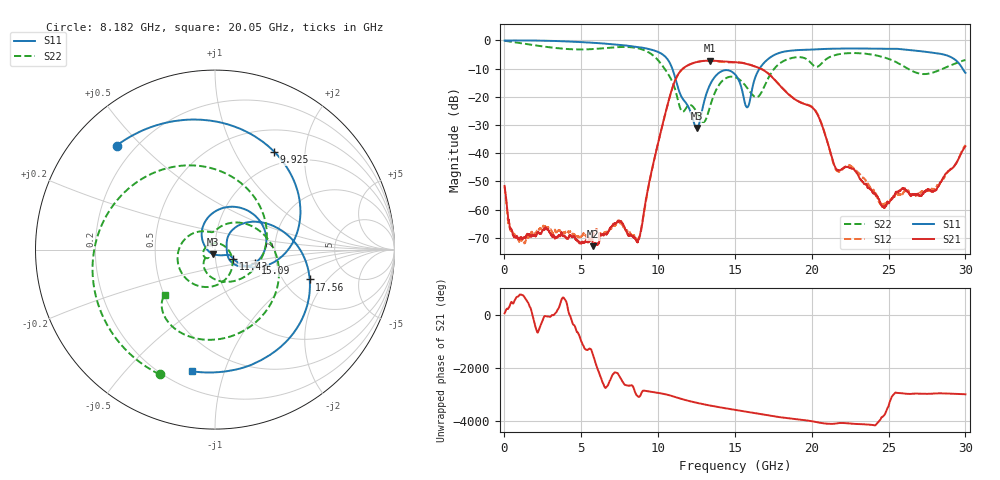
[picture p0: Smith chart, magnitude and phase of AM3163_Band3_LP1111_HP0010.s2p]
!Agilent Technologies,E8364B,MY43040894,A.07.50.67
!Agilent E8364B: A.07.50.67
!Date: Thursday, August 20, 2020 12:15:40
!Correction: S11(Full 2 Port(1,2))
!S21(Full 2 Port(1,2))
!S12(Full 2 Port(1,2))
!S22(Full 2 Port(1,2))
!S2P File: Measurements: S11, S21, S12, S22:
# Hz S  dB  R 50
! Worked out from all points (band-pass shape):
!   3201 points, 10 MHz to 30 GHz, reference 50 ohm
!   highest |S21| = -7.16 dB at 13.38 GHz (marker M1); lowest = -72.9 dB at 5.736 GHz (marker M2)
!   |S21| within 3 dB of the highest: 11.58 GHz to 16.73 GHz (5.157 GHz wide, 36.4 % of centre)
!   lowest |S11| = -31.0 dB at 12.51 GHz (marker M3), VSWR 1.06, Z = 49 - j2.59 ohm
!   |S11| at or under -10 dB: 10.93 GHz to 16.6 GHz (5.674 GHz wide, 41.2 % of centre); 29.81 GHz to end of sweep
!   |S22| runs from -29.0 to -0.1 dB; largest |S21 - S12| = 0.013
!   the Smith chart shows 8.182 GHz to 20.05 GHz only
!   S11 on the Smith chart (normalised r, x): 8.182 GHz: 0.13, +0.42; 9.925 GHz: 0.80, +1.46; 11.43 GHz: 1.22, -0.12; 15.09 GHz: 1.55, -0.25; 17.56 GHz: 2.77, -1.33; 20.05 GHz: 0.30, -0.79
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1e7  -0.04 -2.0  -51.59 49.8  -51.81 -130.8  -0.11 -5.1
1.247088e9  -0.01 -34.1  -70.12 -17.3  -71.29 79.5  -1.12 -82.7
2.652869e9  -0.11 -72.4  -66.44 -54.0  -65.84 103.9  -2.23 -163.0
5.014581e9  -0.60 -135.1  -71.80 53.8  -69.18 113.4  -3.20 71.9
5.736216e9  -0.82 -154.4  -72.94 -31.8  -68.90 -144.7  -3.06 32.0
8.182275e9  -1.96 133.4  -68.85 -162.7  -68.22 59.0  -2.38 -113.9
8.800819e9  -2.41 111.0  -69.56 150.4  -69.26 153.6  -2.91 -157.2
9.925444e9  -3.91 58.8  -38.02 -65.8  -38.02 -65.2  -6.58 98.4
1.000979e10  -4.11 53.9  -36.11 -73.9  -36.10 -73.7  -7.08 87.8
1.143432e10  -18.94 -26.3  -11.00 70.6  -11.04 71.0  -23.96 -138.2
1.251208e10  -31.04 -109.5  -7.66 -89.4  -7.65 -89.0  -25.41 168.1
1.338367e10  -15.63 109.4  -7.16 166.7  -7.19 166.1  -23.37 5.2
1.5005e10  -12.02 -13.2  -7.71 4.1  -7.77 5.8  -13.03 -154.1
1.508935e10  -12.59 -18.7  -7.73 -4.0  -7.77 -2.3  -13.21 -161.3
1.581098e10  -23.69 6.8  -8.37 -73.9  -8.31 -73.2  -16.92 137.2
1.756352e10  -5.14 -17.5  -13.83 116.9  -13.71 117.6  -10.01 5.2
2.000958e10  -3.23 -99.6  -23.66 -65.8  -23.48 -65.5  -8.32 -137.6
2.004707e10  -3.22 -100.5  -23.83 -69.8  -23.63 -69.5  -8.53 -137.9
2.16028e10  -2.91 -137.0  -45.59 -148.9  -45.99 -150.5  -5.07 -160.4
2.500479e10  -2.99 144.8  -57.62 160.0  -57.54 -10.6  -6.55 68.1
2.740399e10  -4.02 77.6  -53.32 -110.7  -53.54 -109.9  -11.91 -88.4
3e10  -11.49 -29.4  -37.52 -128.4  -37.11 -123.6  -6.94 130.5
